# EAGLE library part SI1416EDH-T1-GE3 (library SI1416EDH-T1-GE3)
Si1416EDH-T1-GE3 N-Channel MOSFET, 3.9 A, 30 V, 6-Pin SOT-363 Vishay Source: Datasheet
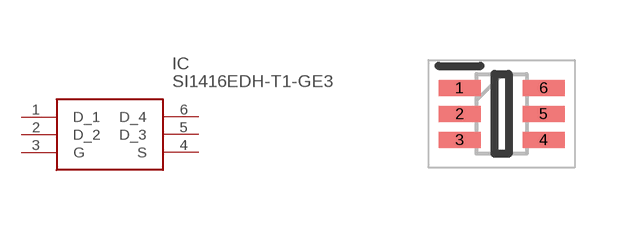
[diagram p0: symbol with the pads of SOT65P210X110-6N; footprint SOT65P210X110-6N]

Designator prefix IC

## SI1416EDH-T1-GE3 (Description: Si1416EDH-T1-GE3 N-Channel MOSFET, 3.9 A, 30 V, 6-Pin SOT-363 Vishay; Height: 1.1mm; Manufacturer_Name: Vishay; Manufacturer_Part_Number: SI1416EDH-T1-GE3; Mouser_Part_Number: 78-SI1416EDH-T1-GE3; Mouser_Price-Stock: https://www.mouser.co.uk/ProductDetail/Vishay-Semiconductors/SI1416EDH-T1-GE3?qs=pNKBmB2EQRiQP6xZUEPceg%3D%3D)  [SOT65P210X110-6N]
1  D_1
2  D_2
3  G
4  S
5  D_3
6  D_4

## Footprint SOT65P210X110-6N (pad centres in mm)
SI1416EDH-T1-GE3-1
smd 1.05 x 0.4: 1 -1.05,0.65; 2 -1.05,0; 3 -1.05,-0.65; 4 1.05,-0.65; 5 1.05,0; 6 1.05,0.65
